FUNCTION_BLOCK FB_Axis
VAR_INPUT
	bDriveReset		: BOOL;				// request reset
	bHalt			: BOOL;				// request stop
	bEnable			: BOOL;				// request enable
	lrVelocity 		: LREAL;			// target velocity
END_VAR
VAR_OUTPUT
	bStatus			: BOOL;				// feedback
	iErrorID		: DWORD;			// error ID
	bMoves			: BOOL;				// status of moving
	bHaltDone		: BOOL;				// status of function block MC_Halt
	bResetDone		: BOOL;				// status of function block MC_Reset
END_VAR
VAR
	lrOverride 		: LREAL := 100.0;	// override 100%
	rtrigHalt		: R_TRIG;
	rtrigReset		: R_TRIG;
	AxisRef			: AXIS_REF;			// axis reference (process data plc/nc)
	fbMcPower 		: MC_Power;			// FB for enable and override
	fbMcReset 		: MC_Reset;			// FB to reset axis
	fbMcStop 		: MC_Stop;			// FB to stop axis
	fbMcHalt		: MC_Halt;			// FB to halt axis
	fbMcMove		: MC_MoveVelocity;	// FB to move axis (velocity movement)
END_VAR

// =========================================================
;
// =========================================================

METHOD PUBLIC M_Stop
VAR_INPUT
END_VAR
// =========================================================

fbMCMove(Execute := FALSE, Axis := AxisRef);
rtrigHalt( CLK := bHalt );

IF rtrigHalt.Q THEN
	bHaltDone := FALSE;
	fbMcStop(Execute := TRUE, Axis := AxisRef);
END_IF

IF NOT rtrigHalt.Q THEN
	fbMcStop(Axis := AxisRef);
END_IF

IF fbMcStop.Done OR fbMcStop.Error OR fbMcStop.CommandAborted THEN
	
	IF fbMcStop.Error THEN
		iErrorID := fbMcStop.ErrorID;
	END_IF
	
	fbMCMove(Execute := FALSE, Axis := AxisRef);
	fbMcStop(Execute := FALSE, Axis := AxisRef);
END_IF

IF NOT fbMcStop.Busy THEN
	bHaltDone := TRUE;
END_IF

// =========================================================
END_METHOD

METHOD PUBLIC M_MoveBw
VAR_INPUT
END_VAR
// =========================================================

IF NOT fbMcMove.Error THEN
	fbMCMove(	Execute := TRUE,
				Velocity := lrVelocity,
				Direction := MC_Negative_Direction,
				Axis := AxisRef );
END_IF

IF fbMCMove.Error OR fbMCMove.CommandAborted THEN
	
	IF fbMcMove.Error THEN
		iErrorID := fbMCMove.ErrorID;
	END_IF
	
	fbMCMove(Execute := FALSE, Axis := AxisRef);
END_IF

// =========================================================
END_METHOD

METHOD PUBLIC M_Enable
VAR_INPUT
END_VAR
// =========================================================

fbMCPower(	Enable 			:= bEnable, 
			Enable_Positive	:= bEnable, 
			Enable_Negative	:= bEnable, 
			Override		:= lrOverride,
			Axis			:= AxisRef,
			Status			=> bStatus	);
			
IF fbMcPower.Error THEN
	iErrorID := fbMcPower.ErrorID;
END_IF

AxisRef.ReadStatus();

bMoves := AxisRef.Status.Moving;

// =========================================================
END_METHOD

METHOD PUBLIC M_Reset
VAR_INPUT
END_VAR
// =========================================================

rtrigReset( CLK := bDriveReset );

IF rtrigReset.Q THEN
	bResetDone := FALSE;
	bHaltDone := FALSE;
	fbMcReset(Execute := TRUE, Axis := AxisRef);
END_IF

fbMcReset(Axis := AxisRef);

IF fbMcReset.Done OR fbMcReset.Error THEN
	iErrorID := fbMcReset.ErrorID;
	
	fbMcReset(Execute := FALSE,	Axis := AxisRef);
	
	bResetDone := TRUE;
END_IF

// =========================================================
END_METHOD

METHOD PUBLIC M_MoveFw
VAR_INPUT
END_VAR
// =========================================================

IF NOT fbMcMove.Error THEN
	fbMCMove(	Execute := TRUE,
				Velocity := lrVelocity,
				Direction := MC_Positive_Direction,
				Axis := AxisRef );
END_IF

IF fbMCMove.Error OR fbMCMove.CommandAborted THEN
	
	IF fbMcMove.Error THEN
		iErrorID := fbMCMove.ErrorID;
	END_IF
	
	fbMCMove(Execute := FALSE, Axis := AxisRef);
END_IF

// =========================================================
END_METHOD

METHOD PUBLIC M_Halt
VAR_INPUT
END_VAR
// =========================================================

fbMCMove(Execute := FALSE, Axis := AxisRef);

rtrigHalt(CLK := bHalt );

IF rtrigHalt.Q THEN
	bHaltDone := FALSE;
	fbMcHalt(Execute := TRUE, Axis := AxisRef);
END_IF

IF NOT rtrigHalt.Q THEN
	fbMcHalt(Axis := AxisRef);
END_IF
	
IF fbMcHalt.Done OR fbMcHalt.Error OR fbMcHalt.CommandAborted THEN
	
	IF fbMcHalt.Error THEN
		iErrorID := fbMcHalt.ErrorID;
	END_IF
	
	fbMCMove(Execute := FALSE, Axis := AxisRef);
	fbMcHalt(Execute := FALSE, Axis := AxisRef);
END_IF

IF NOT fbMcHalt.Busy THEN
	bHaltDone := TRUE;
END_IF

// =========================================================
END_METHOD

END_FUNCTION_BLOCK
